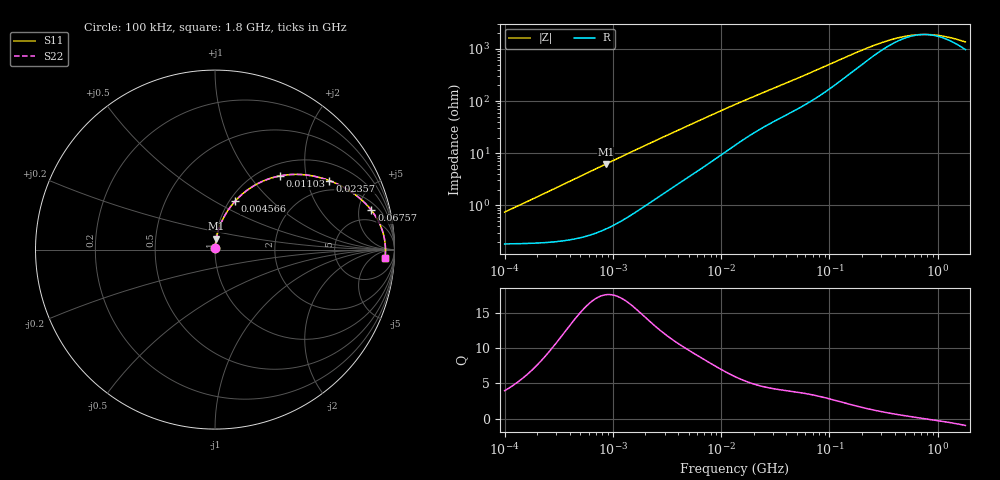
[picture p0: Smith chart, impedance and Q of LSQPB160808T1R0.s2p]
! LSQPB160808T1R0  S-PARAMETER MODEL  ( General Type )
! Model Generated by TAIYO YUDEN Corporation (http://www.ty-top.com)
! Version 4.0
! TAIYO YUDEN Control No. 100810NF18SB-HKC
! Copyright(c) 2007 TAIYO YUDEN CO.,LTD. All Rights Reserved.
! Product Description (link to TY-COMPAS)
! https://ds.yuden.co.jp/TYCOMPAS/or/detail?pn=LSQPB160808T1R0M&u=M
! Products Name : Inductors
! Characteristics :
!  Inductance : 1.0 uH , SRF(min) : 140 MHz , DC Resistance(max) : 0.234 Ohm
!  Rated Current : Saturation :850 mA , Temp Rise : 520 mA (40 degC)
!  Case Size : 1.6 x 0.8 / 0.063 x 0.031 [mm/inch] , Thickness : 0.8 / 0.031 [mm/inch]
!  (Conditions: Temperature = 25 degC , DC Bias Current/Voltage = 0A / 0V)
! External Node Assignments :
!  1  o---GGG---o  2
! GND o---------o GND
! Frequency Range : 0.1MHz  -  1800MHz  [ 402 STEP ]
# MHz S RI R 50
! Freq[MHz].  S11 Real  S11 Imag  S21 Real  S21 Imag  S12 Real  S12 Imag  S22 Real  S22 Imag
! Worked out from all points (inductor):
!   401 points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, 100 kHz to 1.8 GHz, reference 50 ohm
!   read as one part in series: L = 1.15 uH near 105 kHz
!   highest Q = 17.6 at 863.3 kHz (marker M1), where L = 1.14 uH
!   self-resonance near 748 MHz
!   S11 on the Smith chart (normalised r, x): 100 kHz: 1.00, +0.01; 4.566 MHz: 1.06, +0.62; 11.03 MHz: 1.21, +1.42; 23.57 MHz: 1.60, +2.75; 67.57 MHz: 2.99, +6.79; 1.8 GHz: 20, -19
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0.1  0.00187 0.0072  0.9981 -0.0072  0.9981 -0.0072  0.00187 0.0072
0.516129  0.0038 0.037  0.9962 -0.037  0.9962 -0.037  0.0038 0.037
0.863296  0.00732 0.0614  0.9927 -0.0614  0.9927 -0.0614  0.00732 0.0614
1.55409  0.0188 0.1079  0.9812 -0.1079  0.9812 -0.1079  0.0188 0.1079
2.66389  0.0467 0.1753  0.9533 -0.1753  0.9533 -0.1753  0.0467 0.1753
4.566214  0.1111 0.2686  0.8889 -0.2686  0.8889 -0.2686  0.1111 0.2686
6.92477  0.2042 0.348  0.7958 -0.348  0.7958 -0.348  0.2042 0.348
11.02886  0.3598 0.4103  0.6402 -0.4103  0.6402 -0.4103  0.3598 0.4103
13.41641  0.4348 0.4189  0.5652 -0.4189  0.5652 -0.4189  0.4348 0.4189
17.56533  0.5367 0.4117  0.4633 -0.4117  0.4633 -0.4117  0.5367 0.4117
23.56755  0.6373 0.3842  0.3627 -0.3842  0.3627 -0.3842  0.6373 0.3842
39.41996  0.7765 0.3095  0.2235 -0.3095  0.2235 -0.3095  0.7765 0.3095
67.57036  0.8713 0.219  0.1287 -0.219  0.1287 -0.219  0.8713 0.219
69.24595  0.8744 0.215  0.1256 -0.215  0.1256 -0.215  0.8744 0.215
99.99243  0.9103 0.1585  0.0897 -0.1585  0.0897 -0.1585  0.9103 0.1585
151.6408  0.9322 0.1065  0.0678 -0.1065  0.0678 -0.1065  0.9322 0.1065
247.5026  0.9438 0.062  0.0562 -0.062  0.0562 -0.062  0.9438 0.062
357.3983  0.9475 0.0375  0.0525 -0.0375  0.0525 -0.0375  0.9475 0.0375
542.0029  0.9493 0.0153  0.0507 -0.0153  0.0507 -0.0153  0.9493 0.0153
782.6622  0.9498 -0.00211  0.0502 0.00211  0.0502 0.00211  0.9498 -0.00211
1130.179  0.9495 -0.0198  0.0505 0.0198  0.0505 0.0198  0.9495 -0.0198
1800  0.9477 -0.0463  0.0523 0.0463  0.0523 0.0463  0.9477 -0.0463
